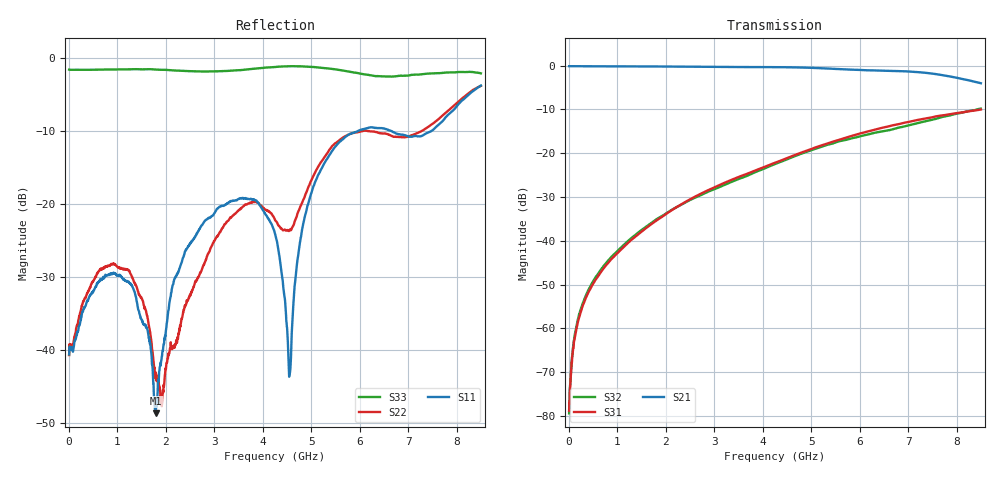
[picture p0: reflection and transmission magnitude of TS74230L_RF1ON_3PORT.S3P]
!Agilent Technologies,E5071C,MY46522130,B.12.04
!Date: Wed Jul 30 10:25:07 2025
!Data & Calibration Information:
!Freq	S11:SOLT3(ON)	S13:SOLT3(ON)	S14:SOLT3(ON)
!	S31:SOLT3(ON)	S33:SOLT3(ON)	S34:SOLT3(ON)
!	S41:SOLT3(ON)	S43:SOLT3(ON)	S44:SOLT3(ON)
!PortZ  Port1:50+j0  Port3:50+j0  Port4:50+j0
!Above PortZ is port z conversion or system Z0 setting when saving the data.
!When reading, reference impedance value at option line is always used.
# Hz S dB R 50
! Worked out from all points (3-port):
!   1601 points, 10 MHz to 8.5 GHz, reference 50 ohm
!   strongest paths, dB at 10 MHz, 2.132 GHz, 4.255 GHz, 6.378 GHz, 8.5 GHz:
!     S21: -0.1, -0.2, -0.4, -1.1, -4.0
!     S31: -78.8, -33.0, -22.2, -14.4, -10.0
!     S32: -79.4, -32.9, -22.5, -15.2, -9.8
!   lowest |S11| = -48.7 dB at 1.798 GHz (marker M1), VSWR 1.01, Z = 50.4 + j0.0805 ohm
!   |S11| at or under -10 dB: start of sweep to 5.984 GHz; 6.633 GHz to 7.492 GHz (858.7 MHz wide, 12.2 % of centre)
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1e7  -40.66 23.9  -0.13 -0.3  -81.40 35.5
     -0.13 -0.3  -40.74 23.0  -77.79 45.9
     -78.81 33.4  -79.39 36.5  -1.64 179.4
3.9205e8  -33.27 66.3  -0.15 -6.6  -52.17 95.3
          -0.15 -6.7  -32.14 50.6  -51.67 92.7
          -52.14 95.1  -51.67 92.7  -1.66 170.3
1.2835e9  -31.08 85.8  -0.18 -21.6  -39.91 106.8
          -0.18 -21.6  -29.72 36.9  -39.48 99.5
          -39.91 106.8  -39.46 99.8  -1.59 151.3
1.798206e9  -48.72 12.6  -0.20 -30.2  -35.49 108.0
            -0.20 -30.3  -43.17 21.8  -35.21 97.5
            -35.46 107.8  -35.19 97.6  -1.63 141.8
2.76925e9  -22.77 -29.5  -0.26 -46.8  -29.02 100.4
           -0.27 -46.9  -28.61 84.7  -29.34 87.4
           -29.01 100.3  -29.34 87.5  -1.90 117.0
4.255e9  -24.11 8.8  -0.35 -73.2  -22.15 82.8
         -0.36 -73.4  -22.21 46.9  -22.49 69.3
         -22.18 82.5  -22.46 69.2  -1.28 87.9
4.557456e9  -43.26 81.2  -0.38 -79.1  -20.92 78.6
            -0.38 -79.2  -23.58 89.7  -21.13 64.0
            -20.88 78.2  -21.15 63.9  -1.18 86.2
4.843994e9  -22.56 -179.0  -0.44 -84.8  -19.72 73.2
            -0.45 -84.9  -19.43 127.4  -19.94 58.1
            -19.68 73.3  -19.91 58.3  -1.21 84.2
5.448906e9  -12.64 -174.2  -0.72 -96.7  -17.38 61.2
            -0.73 -96.9  -12.02 138.2  -17.75 44.0
            -17.37 61.4  -17.76 44.1  -1.56 77.3
8.5e9  -3.82 104.5  -4.03 -160.7  -10.00 -8.8
       -4.02 -161.0  -3.87 77.3  -9.90 -25.8
       -10.02 -8.9  -9.82 -25.0  -2.15 32.7
